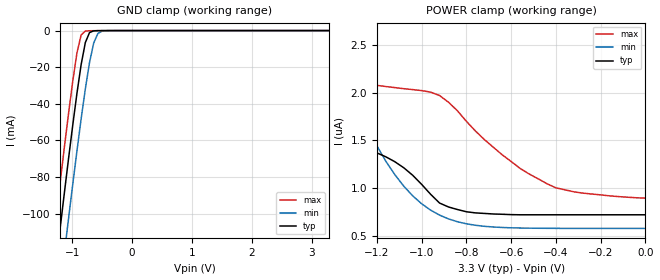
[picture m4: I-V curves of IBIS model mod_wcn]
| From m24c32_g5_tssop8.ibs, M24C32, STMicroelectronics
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|   Model mod_wcn
[Model]   mod_wcn
Model_type Input
Vinl   =   1.000V
Vinh   =   2.300V
C_comp   2.119pF   2.023pF   2.323pF
[Temperature Range]   25.0000   0.1050k   -40.0000
[Voltage Range]   3.3000V   2.7000V   3.6000V
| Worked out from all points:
|   GND clamp passes 1 mA (typ) near -0.70 V on its own axis
[GND_clamp]
|Voltage   I(typ)   I(min)   I(max)
-3.3V     -716.5mA   -747.7mA   -693.4mA
-1.34V    -147mA     -180mA     -122.1mA
-1.27V    -127.4mA   -160.4mA   -102.4mA
-1.2V     -108mA     -141mA     -82.97mA
-1.13V    -88.8mA    -121.7mA   -63.87mA
-1.06V    -69.97mA   -102.7mA   -45.3mA
-920mV    -34.31mA   -65.81mA   -12.26mA
-850mV    -18.61mA   -48.28mA   -2.393mA
-780mV    -6.556mA   -31.87mA   -242.2uA
-640mV    -136.8uA   -6.742mA   -71.43uA
-500mV    -15.34uA   -270.6uA   -32.66uA
3.28V     1.282uA    584.3nA    2.389uA
[POWER_clamp]
|Voltage   I(typ)   I(min)   I(max)
-3.28V    8.547uA    8.769uA    9.331uA
-1.72V    3.569uA    2.634uA    4.042uA
-1.56V    2.649uA    2.397uA    2.8uA
-1.52V    2.39uA     2.338uA    2.601uA
-1.44V    1.969uA    2.217uA    2.318uA
-1.36V    1.669uA    2.086uA    2.167uA
-1.32V    1.56uA     1.997uA    2.127uA
-1.12V    1.277uA    1.142uA    2.051uA
-920mV    844.4nA    718.3nA    1.969uA
-640mV    727nA      588.9nA    1.349uA
-440mV    721.6nA    580.2nA    1.047uA
0V        721.6nA    579nA      895.6nA
